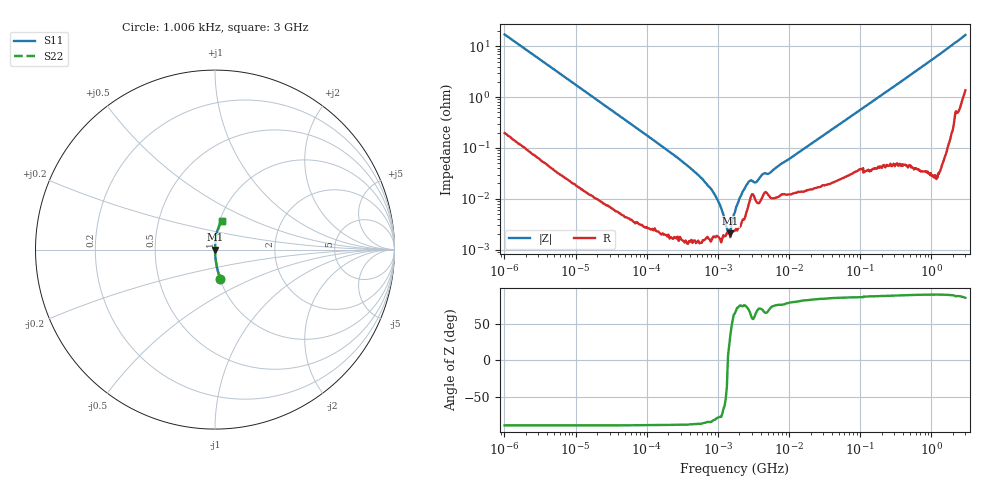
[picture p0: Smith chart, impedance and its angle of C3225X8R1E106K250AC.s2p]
! S-Parameter Data Generated by TDK Corporation
! Copyright(C) 2022 TDK Corporation.
! All Rights Reserved.
! TDK P/N: C3225X8R1E106K250AC (Multilayer Ceramic Chip Capacitor)
! Property: C=10uF
! Size(LxWxT): 3.2x2.5x2.5mm
! Model Type: s2p (Touchstone File Format Version 1.0)
! Frequency: DC=Yes Start=0.00100604MHz Stop=3000MHz 481points Log-sweep
! Model Generated on Apr. 15, 2022
! Port Assignments:
!  1 ---| |--- 2
! Applicable Conditions:
!  Temperature = 25 degC
!  DC Bias Voltage = 0 V
!  Small Signal Operation
! Terms and conditions regarding TDK Simulation Models
! (1)This simulation model is being provided solely for informational purposes. Please refer to the specifications of the products in terms of detailed characteristics of such products.
! (2)In no event shall TDK Corporation of any of its subsidiaries be liable for any loss or damage arising, directly or indirectly,
!  From any information contained in this simulation model, including, but not limited to loss or damages arising from any inaccuracies, omissions or errors in connection with such information.
! (3)Any and all copyrights on this simulation model are owned by TDK Corporation.
!  Duplication or redistribution of this simulation model without prior written permission from TDK Corporation is prohibited.
! (4)This simulation model is subject to any modification or change without any prior notice.
! (5)Neither TDK Corporation nor any of its subsidiaries shall make any warranty, express or implied,
!  Including but not limited to the correctness, implied warranties of merchantability and fitness for a particular purpose with respect to this simulation models.
! (6)The use of this simulation model shall be deemed to have consented to the terms and conditions hereof.
# Hz S MA R 50
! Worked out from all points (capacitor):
!   480 points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, 1.006 kHz to 3 GHz, reference 50 ohm
!   read as one part in series: C = 9.21 uF near 1.083 kHz
!   lowest |Z| = 2.1 mohm at 1.493 MHz (marker M1)
!   series resonance near 1.38 MHz, so ESL is about 1.4 nH
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1006.04  0.1684 -79.6  0.9838 9.7  0.9838 9.7  0.1684 -79.6
2947.59  0.05895 -86.0  0.9976 3.4  0.9976 3.4  0.05895 -86.0
12511.3  0.01407 -88.6  0.9997 0.8  0.9997 0.8  0.01407 -88.6
149930  0.001183 -88.9  1 0.1  1 0.1  0.001183 -88.9
292186  0.0005912 -88.2  1 0.0  1 0.0  0.0005912 -88.2
528729  0.0002942 -87.1  1 0.0  1 0.0  0.0002942 -87.1
765978  0.0001683 -84.6  1 0.0  1 0.0  0.0001683 -84.6
921951  0.000115 -81.3  1 0.0  1 0.0  0.000115 -81.3
992898  9.451e-05 -78.8  1 0.0  1 0.0  9.451e-05 -78.8
1492750  2.096e-05 33.4  1 -0.0  1 -0.0  2.096e-05 33.4
1796710  6.783e-05 67.8  1 -0.0  1 -0.0  6.783e-05 67.8
2008040  0.000102 74.3  1 -0.0  1 -0.0  0.000102 74.3
2508200  0.000185 73.0  0.9999 -0.0  0.9999 -0.0  0.000185 73.0
2803220  0.0002244 66.0  0.9999 -0.0  0.9999 -0.0  0.0002244 66.0
3501450  0.0002157 66.6  0.9999 -0.0  0.9999 -0.0  0.0002157 66.6
4214440  0.0003025 69.1  0.9999 -0.0  0.9999 -0.0  0.0003025 69.1
5462960  0.0003282 71.3  0.9999 -0.0  0.9999 -0.0  0.0003282 71.3
7348770  0.0004613 75.7  0.9999 -0.0  0.9999 -0.0  0.0004613 75.7
2.15311e7  0.001272 83.0  0.9998 -0.1  0.9998 -0.1  0.001272 83.0
2.50734e8  0.01368 87.4  0.9995 -0.8  0.9995 -0.8  0.01368 87.4
1.08091e9  0.05787 86.4  0.998 -3.3  0.998 -3.3  0.05787 86.4
3e9  0.1628 76.0  0.9735 -9.3  0.9735 -9.3  0.1628 76.0
